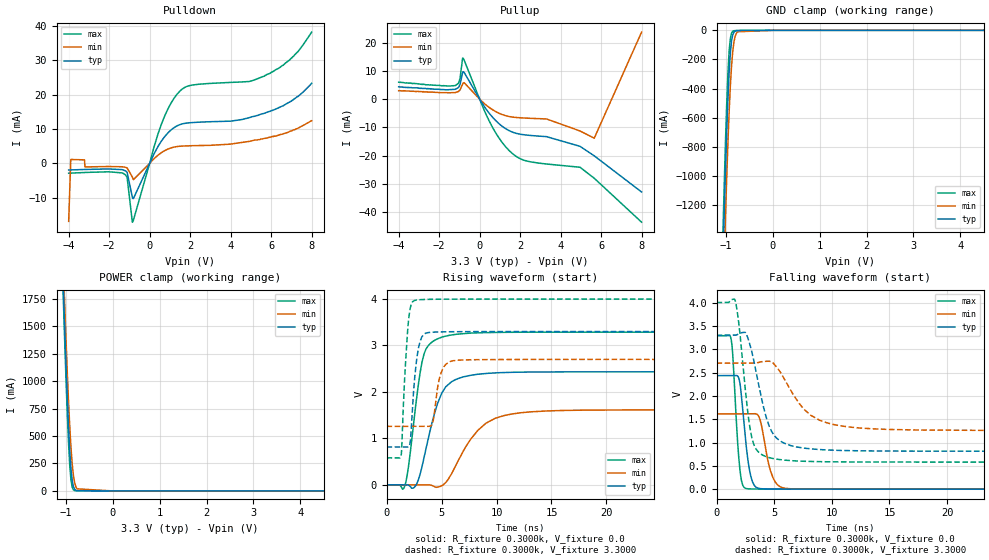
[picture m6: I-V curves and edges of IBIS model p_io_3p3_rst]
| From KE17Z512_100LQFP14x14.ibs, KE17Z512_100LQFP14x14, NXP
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[Model] p_io_3p3_rst
|   Model p_io_3p3_rst
| This model was characterised for following simulation conditions:
| External (pad) voltage:
|   - Typ: 3.3V,   - Min: 2.7V,   - Max: 4.0V
| Library cells for typ/min/max conditions are connected as defined below:
|  pad - External Pad
|  ipp_do_lv - Core Input
|  ipp_obe_lv - Output Buffer Enable
|  abt_close_nor_rst_mv - vdde
|  dvdd - dvdd
|  dvss - dvss
|  esd_boost - vdde
|  ipp_ina_280_mv - NC
|  ipp_ina_40_a_mv - NC
|  ipp_ina_40_b_mv - NC
|  ipp_ina_40_c_mv - NC
|  ipp_ina_40_d_mv - NC
|  ipp_ina_40_e_mv - NC
|  ipp_ina_40_f_mv - NC
|  ipp_ina_40_g_mv - NC
|  ipp_ina_40_h_mv - NC
|  ipp_ind_lv - NC
|  vdde - vdde
|  vsse - vsse
| All other pins connected to ground
Model_type I/O
Polarity   Non-Inverting
Enable   Active-High
Vinl =   0.9900V
Vinh =   2.3100V
Vmeas =  1.6500V
Cref =   50.0000F
C_comp   1.5556pF   1.4873pF   1.6463pF
[Model Spec]
| variable   typ   min   max
Vinh   2.3100V   1.8900V   2.8000V
Vinl   0.9900V   0.8100V   1.2000V
S_overshoot_high   3.6000V   3.0000V   4.3000V
S_overshoot_low   -0.3000V   -0.3000V   -0.3000V
Vmeas   1.6500V   1.3500V   2.0000V
[Temperature Range]   25.0000   0.1250k   -40.0000
[Voltage Range]   3.3000V   2.7000V   4.0000V
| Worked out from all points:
|   slope of the pulldown table from 0 to 0.495 V, typ, clamps not added: 86.9 ohm
|   slope of the pullup table from 0 to 0.495 V, typ, clamps not added: 95.4 ohm
|   rising waveform, R_fixture 0.3000k, V_fixture 0.0: 20-80 % time 1.65ns typ, 2.77ns min, 1.07ns max; typ from 0 V to 2.43 V
|   rising waveform, R_fixture 0.3000k, V_fixture 3.3000: 20-80 % time 534ps typ, 614ps min, 461ps max; typ from 0.814 V to 3.3 V
|   falling waveform, R_fixture 0.3000k, V_fixture 0.0: 20-80 % time 631ps typ, 818ps min, 470ps max; typ from 2.43 V to 0 V
|   falling waveform, R_fixture 0.3000k, V_fixture 3.3000: 20-80 % time 1.45ns typ, 2.67ns min, 898ps max; typ from 3.3 V to 0.814 V
[Pulldown]
|Voltage   I(typ)   I(min)   I(max)
-4V       -1.92mA    -16.86mA   -2.86mA
-3.896V   -1.9mA     1.14mA     -2.83mA
-3.22V    -1.77mA    1.03mA     -2.65mA
-3.194V   -1.76mA    -1.02mA    -2.64mA
-1.192V   -2.171mA   -1.139mA   -3.338mA
-1.114V   -2.581mA   -1.308mA   -4.052mA
-854mV    -9.88mA    -3.961mA   -17.1mA
576mV     6.453mA    3.116mA    11.33mA
1.46V     11.2mA     4.969mA    20.81mA
5.672V    14.6mA     7.3mA      25.4mA
6.92V     17.8mA     9.3mA      30.1mA
8V        23.3mA     12.4mA     38.2mA
[Pullup]
|Voltage   I(typ)   I(min)   I(max)
-4V       4.4mA      3mA        6mA
-1.204V   3.5mA      2.35mA     4.81mA
-970mV    5.149mA    3.27mA     7.302mA
-840mV    9.539mA    5.346mA    14.6mA
486mV     -5.114mA   -3.012mA   -7.929mA
1.058V    -9.302mA   -5.298mA   -14.82mA
1.552V    -11.47mA   -6.274mA   -18.86mA
2.202V    -12.63mA   -6.689mA   -21.68mA
3.3V      -13.29mA   -7.01mA    -22.99mA
4.958V    -16.72mA   -11.28mA   -24.14mA
5.66V     -20.09mA   -13.85mA   -28.04mA
8V        -32.92mA   23.78mA    -43.62mA
[GND_clamp]
|Voltage   I(typ)   I(min)   I(max)
-4V       -44.28A    -44.23A    -44.37A
-1.062V   -1.557A    -1.864A    -1.375A
-1.036V   -1.255A    -1.569A    -1.066A
-1.01V    -970.3mA   -1.287A    -777mA
-958mV    -480.3mA   -781.5mA   -302.1mA
-932mV    -293.3mA   -567.5mA   -146mA
-906mV    -157.3mA   -387.1mA   -56.88mA
-880mV    -73.65mA   -245.3mA   -19.23mA
-828mV    -12.56mA   -78.19mA   -3.038mA
-750mV    -1.35mA    -9.926mA   -1.327mA
0V        -1.644pA   -180pA     -5.223pA
8V        0A         0A         0A
[POWER_clamp]
|Voltage   I(typ)   I(min)   I(max)
-4V       47.58A     47.37A     47.77A
-1.074V   2.105A     2.3A       2.007A
-1.048V   1.765A     1.972A     1.655A
-1.022V   1.437A     1.657A     1.316A
-970mV    837.8mA    1.074A     697.9mA
-918mV    363.6mA    587.5mA    233.2mA
-892mV    200.3mA    395.9mA    99.34mA
-866mV    95.52mA    246.8mA    34.14mA
-814mV    15.78mA    75.64mA    3.24mA
-762mV    2.377mA    18.74mA    589.4uA
0V        66.39pA    869.8pA    65.78pA
8V        0A         0A         0A
[Ramp]
| variable   typ   min   max
dV/dt_r  1.4599/1.6545n   0.9681/2.7719n   1.9724/1.0699n
dV/dt_f  1.4916/1.4484n   0.8648/2.6710n   2.0518/0.8975n
R_load = 0.3000k
[Rising Waveform]
R_fixture= 0.3000k
V_fixture= 0.0
V_fixture_min= 0.0
V_fixture_max= 0.0
|time   V(typ)   V(min)   V(max)
0s        71.43pV    15.79nV    191.2pV
1.619ns   -70.43uV   -613.3nV   -51.18mV
1.96ns    -3.592mV   677.3nV    327.2mV
2.553ns   -48.4mV    108.6nV    1.507V
3.212ns   376.4mV    -62.85uV   2.63V
4.75ns    1.816V     -44.52mV   3.156V
5.883ns   2.216V     226.3mV    3.225V
8.267ns   2.38V      1.164V     3.273V
11.37ns   2.423V     1.524V     3.285V
40ns      2.433V     1.613V     3.287V
[Rising Waveform]
R_fixture= 0.3000k
V_fixture= 3.3000
V_fixture_min= 2.7000
V_fixture_max= 4.0000
|time   V(typ)   V(min)   V(max)
0s        813.9mV    1.259V     580.4mV
1.328ns   814mV      1.259V     630.6mV
1.97ns    815.3mV    1.259V     3.466V
2.178ns   971.5mV    1.259V     3.823V
2.508ns   2.161V     1.259V     3.966V
3.368ns   3.237V     1.259V     3.991V
4.179ns   3.286V     1.323V     3.996V
4.945ns   3.293V     2.4V       3.998V
6.041ns   3.297V     2.671V     3.999V
40ns      3.3V       2.7V       4V
[Falling Waveform]
R_fixture= 0.3000k
V_fixture= 0.0
V_fixture_min= 0.0
V_fixture_max= 0.0
|time   V(typ)   V(min)   V(max)
0s        2.433V     1.613V     3.287V
1.262ns   2.433V     1.613V     3.218V
1.405ns   2.433V     1.613V     2.893V
1.995ns   2.313V     1.613V     490.6mV
2.578ns   915.7mV    1.613V     13.56mV
3.268ns   82.93mV    1.617V     3.145mV
3.781ns   12.04mV    1.485V     1.925mV
4.921ns   2.273mV    230.3mV    828.7uV
5.978ns   1.101mV    17.32mV    464.9uV
40ns      206.8nV    578.5nV    88.49nV
[Falling Waveform]
R_fixture= 0.3000k
V_fixture= 3.3000
V_fixture_min= 2.7000
V_fixture_max= 4.0000
|time   V(typ)   V(min)   V(max)
0s        3.3V       2.7V       4V
1.619ns   3.3V       2.7V       4.042V
1.984ns   3.339V     2.7V       3.444V
2.499ns   3.359V     2.7V       2.129V
2.998ns   3.004V     2.7V       1.179V
4.441ns   1.442V     2.743V     685mV
5.478ns   1.04V      2.529V     633.9mV
8.169ns   863.8mV    1.584V     593.1mV
10.86ns   829.2mV    1.353V     584mV
40ns      813.9mV    1.259V     580.4mV
